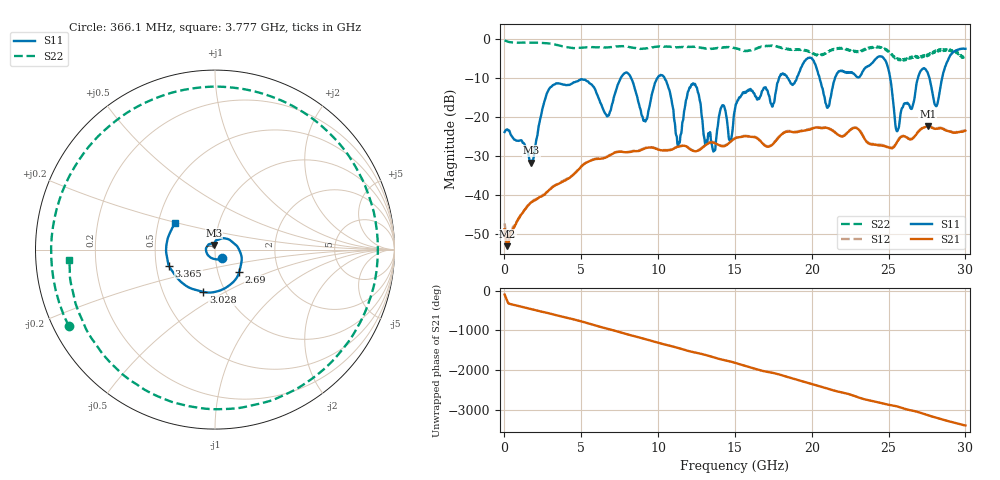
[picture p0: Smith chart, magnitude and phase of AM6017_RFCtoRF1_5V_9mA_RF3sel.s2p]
!Agilent Technologies,E8364B,MY43040894,A.07.50.67
!Agilent E8364B: A.07.50.67
!Date: Tuesday, August 21, 2018 13:34:24
!Correction: S11(Full 2 Port(1,2))
!S21(Full 2 Port(1,2))
!S12(Full 2 Port(1,2))
!S22(Full 2 Port(1,2))
!S2P File: Measurements: S11, S21, S12, S22:
# Hz S  dB  R 50
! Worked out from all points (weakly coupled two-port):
!   1601 points, 10 MHz to 30 GHz, reference 50 ohm
!   highest |S21| = -22.35 dB at 27.54 GHz (marker M1); lowest = -53.1 dB at 178.7 MHz (marker M2)
!   lowest |S11| = -31.6 dB at 1.753 GHz (marker M3), VSWR 1.05, Z = 49.3 + j2.51 ohm
!   |S11| at or under -10 dB: start of sweep to 7.558 GHz; 10.42 GHz to 17.86 GHz (7.437 GHz wide, 52.6 % of centre); 25.11 GHz to 26.9 GHz (1.795 GHz wide, 6.9 % of centre)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
!   |S22| runs from -5.6 to -0.3 dB; largest |S21 - S12| = 0.0053
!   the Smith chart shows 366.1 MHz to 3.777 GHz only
!   S11 on the Smith chart (normalised r, x): 366.1 MHz: 1.08, -0.11; 2.69 GHz: 1.27, -0.32; 3.028 GHz: 0.79, -0.40; 3.365 GHz: 0.58, -0.11; 3.777 GHz: 0.62, +0.19
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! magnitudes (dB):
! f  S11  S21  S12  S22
! 10 MHz  -23.8  -48.8  -47.3  -0.3
! 178.7 MHz  -23.1  -53.1  -52.5  -0.5
! 366.1 MHz  -24.0  -50.2  -50.4  -0.7
! 1.753 GHz  -31.6  -41.8  -41.9  -0.8
! 2.69 GHz  -14.7  -39.5  -39.5  -1.0
! 3.028 GHz  -12.2  -38.4  -38.2  -1.1
! 3.365 GHz  -11.3  -37.4  -37.3  -1.4
! 3.777 GHz  -11.5  -36.6  -36.4  -1.8
! 5.015 GHz  -10.2  -32.6  -32.6  -2.1
! 9.157 GHz  -21.1  -28.0  -27.9  -2.3
! 10.02 GHz  -9.5  -28.3  -28.2  -1.9
! 11.31 GHz  -27.1  -27.6  -27.4  -2.1
! 12.27 GHz  -11.3  -28.6  -28.5  -2.0
! 13.6 GHz  -28.8  -26.5  -26.4  -2.4
! 15.01 GHz  -17.8  -25.4  -25.3  -2.3
! 20.01 GHz  -4.9  -23.0  -22.9  -3.3
! 21.02 GHz  -17.6  -22.8  -22.6  -3.4
! 25.01 GHz  -8.1  -27.8  -27.7  -3.1
! 25.58 GHz  -23.6  -26.2  -26.1  -4.8
! 27.54 GHz  -8.6  -22.3  -22.2  -4.1
! 28.11 GHz  -17.2  -22.9  -22.8  -3.3
! 30 GHz  -2.4  -23.5  -23.4  -5.6
